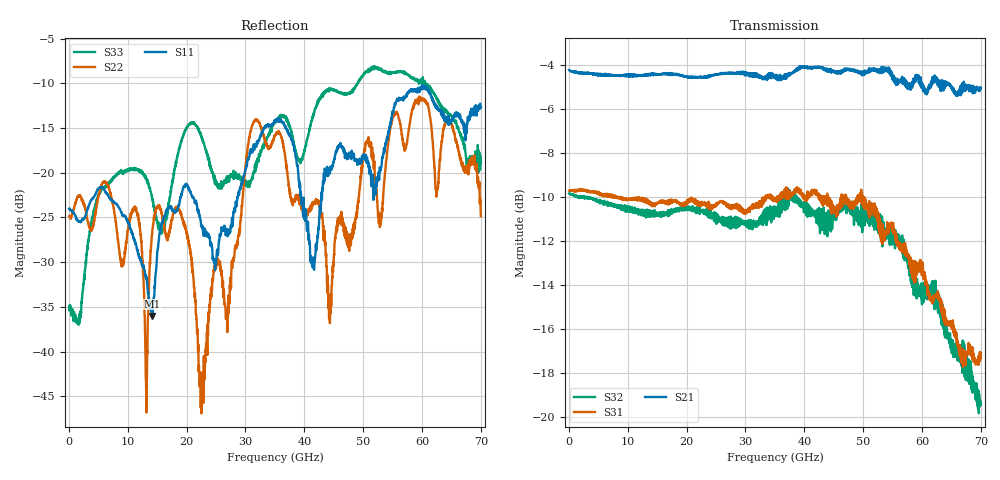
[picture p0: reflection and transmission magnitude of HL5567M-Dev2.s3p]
! 2/10/2020 1:45:37 PM
! H:\PROTOTYPE_DATA\HL9467M\LA01B.S3P
! CHANNEL.1
! TR.MEASUREMENT
! CORRECTED.DATA
# GHZ S RI R 50.0
! FREQ.GHZ  S11RE  S11IM  S12RE  S12IM  S13RE  S13IM
!  S21RE  S21IM  S22RE  S22IM  S23RE  S23IM
!  S31RE  S31IM  S32RE  S32IM  S33RE  S33IM
!; PortSelection: Port_123
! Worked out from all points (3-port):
!   2000 points, 35 MHz to 70 GHz, reference 50 ohm
!   strongest paths, dB at 35 MHz, 17.54 GHz, 35.03 GHz, 52.53 GHz, 70 GHz:
!     S21: -4.2, -4.5, -4.5, -4.3, -5.1
!     S31: -9.7, -10.1, -10.1, -11.0, -17.1
!     S32: -9.8, -10.6, -10.8, -11.0, -19.4
!   lowest |S11| = -36.0 dB at 14.14 GHz (marker M1), VSWR 1.03, Z = 50.9 - j1.33 ohm
!   |S11| at or under -10 dB: start of sweep to end of sweep
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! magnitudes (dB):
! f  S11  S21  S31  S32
! 35 MHz  -24.0  -4.2  -9.7  -9.8
! 11.41 GHz  -28.0  -4.5  -10.1  -10.6
! 13.16 GHz  -31.9  -4.5  -10.1  -10.6
! 14.14 GHz  -36.0  -4.5  -10.3  -10.8
! 19.21 GHz  -22.2  -4.5  -10.4  -10.5
! 22.5 GHz  -26.0  -4.6  -10.4  -10.6
! 35.03 GHz  -14.3  -4.5  -10.1  -10.8
! 44.31 GHz  -20.0  -4.3  -10.4  -11.0
! 55.44 GHz  -12.4  -4.8  -11.6  -11.8
! 70 GHz  -12.7  -5.1  -17.1  -19.4
